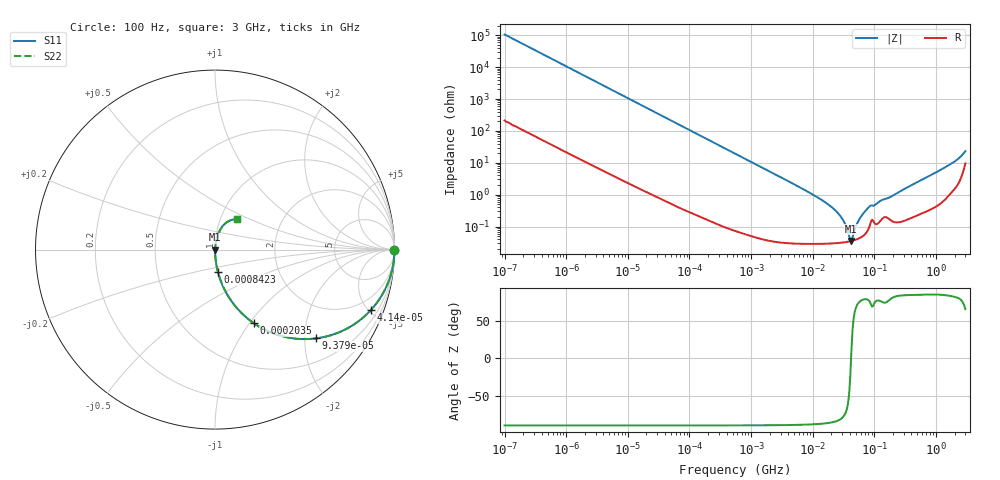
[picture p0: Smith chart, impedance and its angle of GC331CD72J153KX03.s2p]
!Murata Part Number: GC331CD72J153KX03
!These Parameters are Measured in Series Mode Connection
!Data Generated on Jan 08, 2026
!  o--ll--o
!Port1  Port2
!  o------o
!Operation Temp=25[degC], DC Bias Voltage=0[V]
!Freq. Start=100[Hz] Stop=3[GHz] 401[Steps]
# Hz S RI R 50
!Freq.(Hz) S11(Real) S11(Imag) S21(Real) S21(Imag) S12(Real) S12(Imag) S22(Real) S22(Imag)
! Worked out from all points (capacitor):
!   401 points, 100 Hz to 3 GHz, reference 50 ohm
!   read as one part in series: C = 15.1 nF near 109 Hz
!   lowest |Z| = 35.7 mohm at 42.32 MHz (marker M1)
!   series resonance near 41.92 MHz, so ESL is about 960 pH
!   S11 on the Smith chart (normalised r, x): 100 Hz: open; 41.4 kHz: 1.01, -5.15; 93.79 kHz: 1.01, -2.27; 203.5 kHz: 1.00, -1.05; 842.3 kHz: 1.00, -0.25; 3 GHz: 1.19, +0.42
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100  1 -0.000946  2.8e-06 0.000946  2.8e-06 0.000946  1 -0.000946
1788  0.9997 -0.0169  0.000318 0.0169  0.000318 0.0169  0.9997 -0.0169
9582  0.9918 -0.0894  0.00825 0.0894  0.00825 0.0894  0.9918 -0.0894
31977  0.9168 -0.2751  0.0832 0.2751  0.0832 0.2751  0.9168 -0.2751
41399  0.8682 -0.3371  0.1318 0.3371  0.1318 0.3371  0.8682 -0.3371
93790  0.5638 -0.4946  0.4362 0.4946  0.4362 0.4946  0.5638 -0.4946
203529  0.2166 -0.4105  0.7834 0.4105  0.7834 0.4105  0.2166 -0.4105
547723  0.0374 -0.1878  0.9626 0.1878  0.9626 0.1878  0.0374 -0.1878
842342  0.0164 -0.1249  0.9836 0.1249  0.9836 0.1249  0.0164 -0.1249
9794414  0.000393 -0.0103  0.9996 0.0103  0.9996 0.0103  0.000393 -0.0103
1.713898e7  0.000318 -0.00522  0.9997 0.00522  0.9997 0.00522  0.000318 -0.00522
2.52476e7  0.000311 -0.00271  0.9997 0.00271  0.9997 0.00271  0.000311 -0.00271
3.131008e7  0.00032 -0.00152  0.9997 0.00152  0.9997 0.00152  0.00032 -0.00152
3.882828e7  0.00034 -0.000395  0.9997 0.000395  0.9997 0.000395  0.00034 -0.000395
4.231884e7  0.000353 5.04e-05  0.9996 -5.04e-05  0.9996 -5.04e-05  0.000353 5.04e-05
4.418008e7  0.000361 0.000274  0.9996 -0.000274  0.9996 -0.000274  0.000361 0.000274
5.719833e7  0.000435 0.00166  0.9996 -0.00166  0.9996 -0.00166  0.000435 0.00166
7.730952e7  0.000739 0.00357  0.9993 -0.00357  0.9993 -0.00357  0.000739 0.00357
1.295826e8  0.00166 0.00642  0.9983 -0.00642  0.9983 -0.00642  0.00166 0.00642
1.751444e8  0.00176 0.00793  0.9982 -0.00793  0.9982 -0.00793  0.00176 0.00793
1.642185e9  0.0167 0.0834  0.9833 -0.0834  0.9833 -0.0834  0.0167 0.0834
3e9  0.1206 0.1703  0.8794 -0.1703  0.8794 -0.1703  0.1206 0.1703
